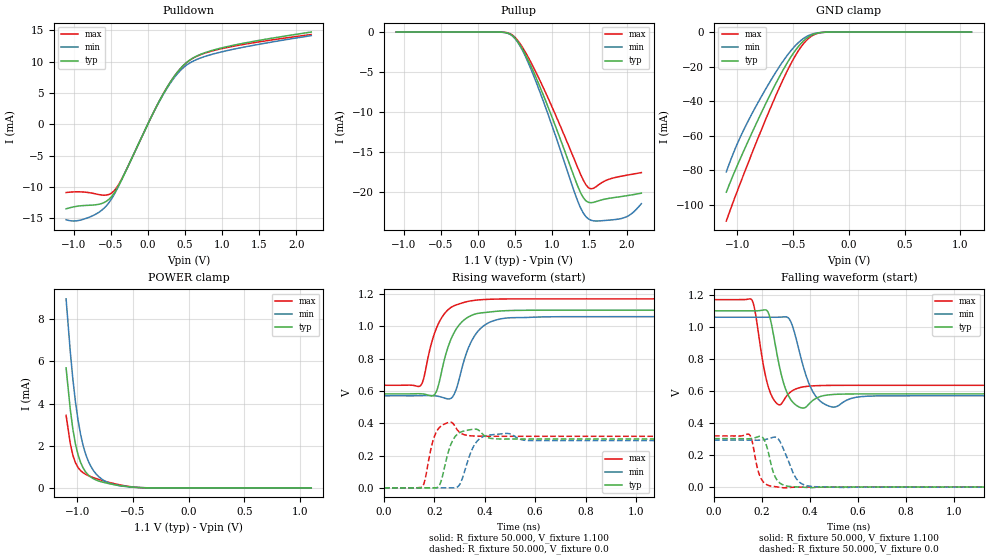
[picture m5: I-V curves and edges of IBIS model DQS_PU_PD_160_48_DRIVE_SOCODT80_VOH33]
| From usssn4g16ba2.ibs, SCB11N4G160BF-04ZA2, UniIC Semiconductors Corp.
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|   Model DQS_PU_PD_160_48_DRIVE_SOCODT80_VOH33
[Model] DQS_PU_PD_160_48_DRIVE_SOCODT80_VOH33
Model_type I/O
Polarity   Inverting
Vinl =  98.000mV
Vinh =  0.268V
Vmeas =  0.183V
Rref =  50.000
Vref =  0.183V
C_comp   1.020pF   1.010pF   1.030pF
[Model Spec]
Vinh   0.268V   0.262V   0.280V
Vinl   98.000mV   92.000mV   0.110V
Vmeas   0.183V   0.177V   0.195V
Vref   0.183V   0.177V   0.195V
Rref   50.000   NA   NA
[Temperature Range]   25.000   0.105k   -40.000
[Voltage Range]   1.100V   1.060V   1.170V
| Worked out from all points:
|   slope of the pulldown table from 0 to 0.165 V, typ, clamps not added: 42.3 ohm
|   GND clamp passes 1 mA (typ) near -0.30 V on its own axis
|   POWER clamp passes 1 mA (typ) near -0.95 V on its own axis
|   rising waveform, R_fixture 50.000, V_fixture 1.100: 20-80 % time 68.4ps typ, 71.6ps min, 66.4ps max; typ from 0.582 V to 1.1 V
|   rising waveform, R_fixture 50.000, V_fixture 0.0: 20-80 % time 29.2ps typ, 37.6ps min, 23.7ps max; typ from 0 V to 0.302 V
|   falling waveform, R_fixture 50.000, V_fixture 1.100: 20-80 % time 41.2ps typ, 54.4ps min, 33.2ps max; typ from 1.1 V to 0.582 V
|   falling waveform, R_fixture 50.000, V_fixture 0.0: 20-80 % time 34ps typ, 50.3ps min, 29.5ps max; typ from 0.302 V to 0 V
[Pulldown]
|Voltage   I(typ)   I(min)   I(max)
-1.1V     -13.51mA   -15.24mA   -10.91mA
-930mV    -13.06mA   -15.37mA   -10.79mA
-726mV    -12.89mA   -14.52mA   -11.06mA
-556mV    -12.29mA   -13.01mA   -11.31mA
-454mV    -11.04mA   -11.25mA   -10.65mA
-318mV    -8.03mA    -8.027mA   -7.964mA
158mV     3.751mA    3.687mA    3.768mA
328mV     7.153mA    6.973mA    7.158mA
498mV     9.598mA    9.214mA    9.581mA
668mV     10.93mA    10.37mA    10.89mA
940mV     12.01mA    11.39mA    11.91mA
2.2V      14.71mA    14.14mA    14.31mA
[Pullup]
|Voltage   I(typ)   I(min)   I(max)
-1.1V     1.606nA    16.44nA    0A
296mV     -8.845uA   -14.64uA   -4.922uA
466mV     -464.7uA   -507.7uA   -387.5uA
568mV     -1.641mA   -1.758mA   -1.466mA
738mV     -4.764mA   -5.196mA   -4.236mA
976mV     -10.14mA   -11.16mA   -8.932mA
1.316V    -18.65mA   -20.49mA   -16.37mA
1.452V    -21.12mA   -23.1mA    -19.11mA
1.554V    -21.33mA   -23.64mA   -19.57mA
1.928V    -20.6mA    -23.36mA   -18.06mA
2.064V    -20.4mA    -22.78mA   -17.83mA
2.2V      -20.18mA   -21.49mA   -17.6mA
[GND_clamp]
|Voltage   I(typ)   I(min)   I(max)
-1.1V     -92.78mA   -81.05mA   -109.5mA
-1.031V   -81.73mA   -69.22mA   -97.17mA
-939mV    -68.18mA   -56.02mA   -81.64mA
-824mV    -52mA      -41.83mA   -62.83mA
-686mV    -33.62mA   -26.41mA   -41.32mA
-571mV    -19.76mA   -15.06mA   -24.85mA
-479mV    -10.5mA    -7.76mA    -13.5mA
-410mV    -5.313mA   -3.84mA    -6.916mA
-341mV    -2.007mA   -1.45mA    -2.59mA
-272mV    -506.9uA   -403.5uA   -609.8uA
-180mV    -45.65uA   -51.35uA   -43.55uA
1.1V      0A         0A         0A
[POWER_clamp]
|Voltage   I(typ)   I(min)   I(max)
-1.1V     5.691mA    8.967mA    3.44mA
-1.062V   3.709mA    6.444mA    2.092mA
-1.039V   2.781mA    5.152mA    1.546mA
-1.016V   2.086mA    4.085mA    1.193mA
-970mV    1.21mA     2.539mA    818.5uA
-947mV    943.7uA    2.005mA    716.7uA
-901mV    610.1uA    1.27mA     581.3uA
-855mV    430.7uA    824.1uA    484.6uA
-786mV    289.9uA    439.4uA    366uA
-671mV    155.9uA    155.9uA    203.6uA
-441mV    13.2uA     12.79uA    15.03uA
1.1V      0A         0A         0A
[Ramp]
| variable   typ   min   max
dV/dt_r   0.181/29.058p   0.176/37.656p   0.192/23.828p
dV/dt_f   0.311/41.295p   0.294/54.417p   0.321/33.258p
R_load = 50.000
[Rising Waveform]
R_fixture= 50.000
V_fixture= 1.100
V_fixture_min= 1.060
V_fixture_max= 1.170
|time   V(typ)   V(min)   V(max)
0s        581.6mV    569.9mV    635mV
148ps     582.3mV    570.6mV    638.1mV
208ps     596.2mV    568.9mV    987.6mV
267ps     923.9mV    555.2mV    1.118V
286ps     981.5mV    606.5mV    1.132V
309ps     1.027V     738.3mV    1.144V
367ps     1.078V     957.8mV    1.162V
445ps     1.093V     1.04V      1.169V
645ps     1.1V       1.059V     1.17V
3ns       1.1V       1.06V      1.17V
[Rising Waveform]
R_fixture= 50.000
V_fixture= 0.0
V_fixture_min= 0.0
V_fixture_max= 0.0
|time   V(typ)   V(min)   V(max)
0s        2.898uV    10.6uV     684.5nV
152ps     91.82uV    31.04uV    6.559mV
196ps     379.1uV    80.29uV    299.2mV
218ps     10.32mV    250.2uV    369.7mV
263ps     258.7mV    111.1uV    406.7mV
302ps     343.2mV    24.53mV    341.9mV
375ps     357.5mV    297.9mV    319.9mV
483ps     302.1mV    336.8mV    319.2mV
579ps     302.1mV    292.7mV    319.2mV
3ns       302.1mV    293.3mV    319.2mV
[Falling Waveform]
R_fixture= 50.000
V_fixture= 1.100
V_fixture_min= 1.060
V_fixture_max= 1.170
|time   V(typ)   V(min)   V(max)
0s        1.1V       1.06V      1.17V
157ps     1.1V       1.06V      1.169V
225ps     1.092V     1.06V      630.9mV
270ps     770.6mV    1.06V      513.5mV
314ps     559.4mV    1.048V     587.1mV
348ps     504.9mV    890.5mV    616.4mV
411ps     540.2mV    596.7mV    631.5mV
497ps     577.9mV    499.2mV    634.6mV
681ps     581.5mV    568.9mV    635mV
3ns       581.6mV    569.9mV    635mV
[Falling Waveform]
R_fixture= 50.000
V_fixture= 0.0
V_fixture_min= 0.0
V_fixture_max= 0.0
|time   V(typ)   V(min)   V(max)
0s        302.1mV    293.3mV    319.2mV
147ps     301.6mV    292.8mV    327.4mV
182ps     313.4mV    292.3mV    109.6mV
199ps     314.2mV    293.5mV    44.9mV
217ps     265.7mV    298mV      17.3mV
252ps     72.44mV    311.8mV    2.954mV
287ps     13.72mV    245mV      -4.393mV
343ps     1.175mV    51.85mV    -677.5uV
413ps     -3.05mV    2.942mV    -18.39uV
3ns       -1.2uV     10.58uV    87.87nV
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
